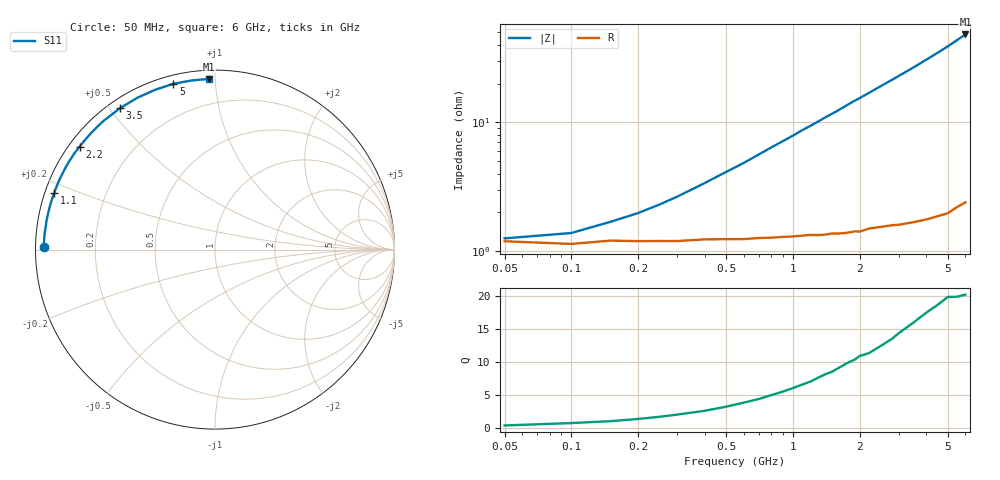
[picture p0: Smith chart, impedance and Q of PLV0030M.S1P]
! Infineon Technologies  Discrete & RF Semiconductors
! BAR 64-04W /-05W /-06W
! Si PIN Diode in SOT323
! IF = 30 mA
! S-Parameters:  October  2008
# GHz  S  MA  R  50
!  f  S11
! GHz  MAG  ANG
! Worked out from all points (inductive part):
!   34 points, 50 MHz to 6 GHz, reference 50 ohm
!   read as one part to ground: L = 1.24 nH near 500 MHz
!   highest Q = 20.2 at 6 GHz (marker M1), where L = 1.28 nH
!   S11 on the Smith chart (normalised r, x): 50 MHz: 0.02, +0.01; 1.1 GHz: 0.03, +0.17; 2.2 GHz: 0.03, +0.34; 3.5 GHz: 0.03, +0.53; 5 GHz: 0.04, +0.78; 6 GHz: 0.05, +0.96
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0.05  0.9535 179.1
0.1  0.9556 178.2
0.15  0.953 177.3
0.2  0.9534 176.4
0.3  0.9534 174.6
0.5  0.952 171.0
0.6  0.9521 169.3
0.8  0.9512 165.7
1  0.9506 162.3
1.1  0.9501 160.5
1.2  0.9498 158.9
1.3  0.9501 157.2
1.4  0.95 155.5
1.6  0.9498 152.3
1.8  0.9495 148.9
1.9  0.9489 147.3
2  0.9495 145.8
2.2  0.9477 142.7
2.4  0.9477 139.6
2.6  0.9477 136.6
2.8  0.9478 133.7
3  0.9485 130.8
3.5  0.9492 123.8
4  0.9502 116.9
4.5  0.9509 110.4
5  0.9522 104.1
5.5  0.9513 97.9
6  0.9517 92.1
